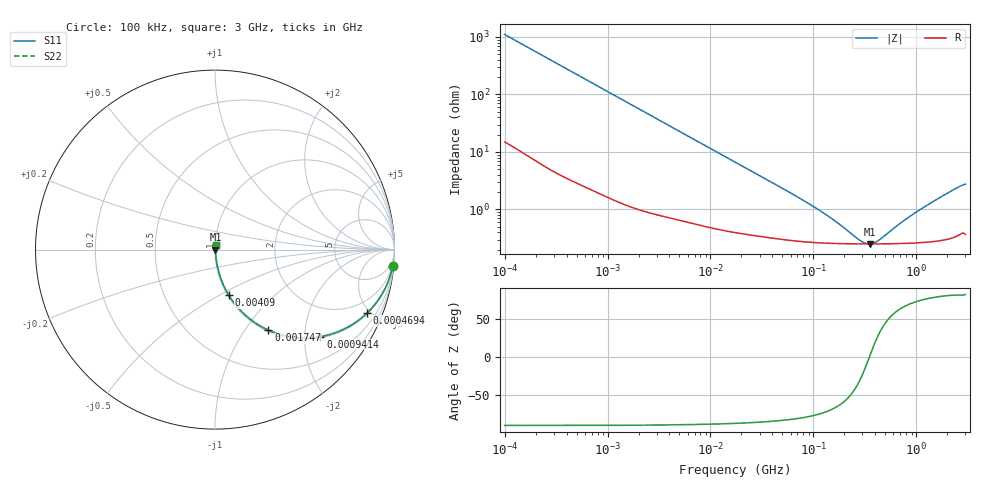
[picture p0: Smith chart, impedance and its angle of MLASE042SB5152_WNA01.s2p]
! MLASE042SB5152_WNA01  S-PARAMETER MODEL  ( Standard Model )
! Model Generated by TAIYO YUDEN Corporation (http://www.ty-top.com)
! Version 1.0
! TAIYO YUDEN Control No. 220601
! Copyright(c) 2016 TAIYO YUDEN CO.,LTD. All Rights Reserved.
! Product Description (link to TY-COMPAS)
! https://ds.yuden.co.jp/TYCOMPAS/or/detail?pn=MLASE042SB5152KWNA01&u=M
! Products Name : Multilayer Ceramic Capacitors
! Characteristics :
!  Capacitance : 1500 [pF] , Rated Voltage : 16 [V] , TCC : X5R
!  Case Size : 0.4 x 0.2 / 0.016 x 0.008 [mm/inch] , Thickness : 0.2 / 0.008 [mm/inch]
!  (Conditions: Temperature = 25 [degC] , DC Bias Voltage = 0 [V])
! External Node Assignments :
!  1  o---| |---o  2
! GND o---------o GND
! Frequency Range : 100kHz  -  3GHz  [ 401 STEP ]
# MHZ S RI R 50
! Freq[MHz].  S11 Real  S11 Imag  S21 Real  S21 Imag  S12 Real  S12 Imag  S22 Real  S22 Imag
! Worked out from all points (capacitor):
!   401 points, 100 kHz to 3 GHz, reference 50 ohm
!   read as one part in series: C = 1.44 nF near 105.3 kHz
!   lowest |Z| = 252 mohm at 353.3 MHz (marker M1)
!   series resonance near 349.1 MHz, so ESL is about 140 pH
!   S11 on the Smith chart (normalised r, x): 100 kHz: 1, -22; 469.4 kHz: 1.06, -4.77; 941.4 kHz: 1.03, -2.39; 1.747 MHz: 1.02, -1.29; 4.09 MHz: 1.01, -0.56; 3 GHz: 1.01, +0.05
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0.1  0.9907 -0.0895  0.0093 0.0895  0.0093 0.0895  0.9907 -0.0895
0.252895  0.9487 -0.2146  0.0513 0.2146  0.0513 0.2146  0.9487 -0.2146
0.469427  0.8472 -0.3535  0.1528 0.3535  0.1528 0.3535  0.8472 -0.3535
0.562235  0.7958 -0.3966  0.2042 0.3966  0.2042 0.3966  0.7958 -0.3966
0.941399  0.5869 -0.4853  0.4131 0.4853  0.4131 0.4853  0.5869 -0.4853
1.282589  0.4368 -0.4884  0.5632 0.4884  0.5632 0.4884  0.4368 -0.4884
1.747435  0.2978 -0.449  0.7022 0.449  0.7022 0.449  0.2978 -0.449
2.320182  0.1967 -0.3882  0.8033 0.3882  0.8033 0.3882  0.1967 -0.3882
3.161081  0.1194 -0.3134  0.8806 0.3134  0.8806 0.3134  0.1194 -0.3134
4.09038  0.0773 -0.2546  0.9227 0.2546  0.9227 0.2546  0.0773 -0.2546
8.202936  0.0241 -0.1356  0.9759 0.1356  0.9759 0.1356  0.0241 -0.1356
17.7727  0.00808 -0.0643  0.9919 0.0643  0.9919 0.0643  0.00808 -0.0643
97.38194  0.00279 -0.0112  0.9972 0.0112  0.9972 0.0112  0.00279 -0.0112
158.9065  0.00259 -0.00594  0.9974 0.00594  0.9974 0.00594  0.00259 -0.00594
287.4592  0.00251 -0.00134  0.9975 0.00134  0.9975 0.00134  0.00251 -0.00134
353.2796  0.00251 8.16e-05  0.9975 -8.16e-05  0.9975 -8.16e-05  0.00251 8.16e-05
423.1245  0.00251 0.00132  0.9975 -0.00132  0.9975 -0.00132  0.00251 0.00132
547.5153  0.00254 0.00318  0.9975 -0.00318  0.9975 -0.00318  0.00254 0.00318
785.4083  0.0026 0.00616  0.9974 -0.00616  0.9974 -0.00616  0.0026 0.00616
1186.261  0.00278 0.0106  0.9972 -0.0106  0.9972 -0.0106  0.00278 0.0106
2378.954  0.00382 0.0224  0.9962 -0.0224  0.9962 -0.0224  0.00382 0.0224
3000  0.00439 0.0271  0.9956 -0.0271  0.9956 -0.0271  0.00439 0.0271
